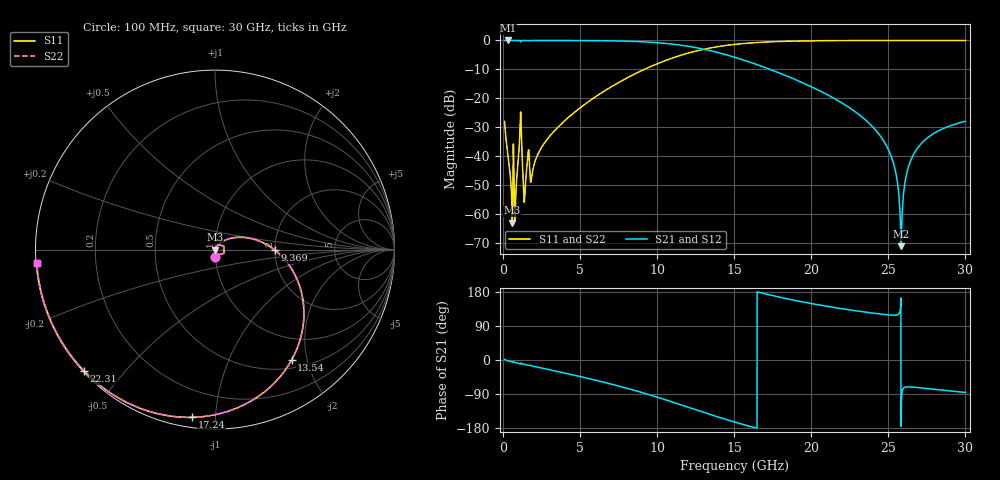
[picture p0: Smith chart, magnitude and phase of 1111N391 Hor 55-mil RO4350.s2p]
# GHz S MA R 50
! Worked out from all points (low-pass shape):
!   3201 points, 100 MHz to 30 GHz, reference 50 ohm
!   highest |S21| = 0.00 dB at 305.6 MHz (marker M1); lowest = -71.2 dB at 25.83 GHz (marker M2)
!   |S21| within 3 dB of the highest: start of sweep to 13 GHz
!   lowest |S11| = -63.1 dB at 595.2 MHz (marker M3), VSWR 1.00, Z = 50.1 - j0.0355 ohm
!   |S11| at or under -10 dB: start of sweep to 9.173 GHz
!   |S22| runs from -63.1 to 0.0 dB; largest |S21 - S12| = 0
!   S11 on the Smith chart (normalised r, x): 100 MHz: 1.00, -0.08; 9.369 GHz: 2.00, -0.01; 13.54 GHz: 0.62, -1.74; 17.24 GHz: 0.05, -0.87; 22.31 GHz: 0.00, -0.39; 30 GHz: 0.00, -0.04
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0.1  0.03985 -88.2  0.9989 1.5  0.9989 1.5  0.03985 -88.2
0.3055625  0.01083 -90.0  0.9995 -1.9  0.9995 -1.9  0.01083 -90.0
0.5952188  0.0006979 -30.5  0.9993 -4.8  0.9993 -4.8  0.0006979 -30.5
0.8661875  0.003414 69.9  0.9991 -7.3  0.9991 -7.3  0.003414 69.9
1.099781  0.02979 54.7  0.987 -10.5  0.987 -10.5  0.02979 54.7
1.417469  0.002259 36.9  0.9983 -11.6  0.9983 -11.6  0.002259 36.9
1.604344  0.01011 46.7  0.9948 -13.6  0.9948 -13.6  0.01011 46.7
1.875312  0.004699 52.9  0.998 -15.5  0.998 -15.5  0.004699 52.9
2.781656  0.0182 63.3  0.9985 -23.5  0.9985 -23.5  0.0182 63.3
5.089563  0.07116 44.5  0.9956 -44.4  0.9956 -44.4  0.07116 44.5
9.369  0.334 -0.5  0.9391 -90.1  0.9391 -90.1  0.334 -0.5
10.06978  0.4013 -9.2  0.9121 -98.9  0.9121 -98.9  0.4013 -9.2
13.53631  0.7488 -55.2  0.6569 -144.9  0.6569 -144.9  0.7488 -55.2
15.05  0.8559 -74.2  0.51 -163.9  0.51 -163.9  0.8559 -74.2
17.23644  0.9433 -97.8  0.3222 172.5  0.3222 172.5  0.9433 -97.8
20.03956  0.9849 -121.6  0.1563 148.7  0.1563 148.7  0.9849 -121.6
22.31009  0.9947 -137.1  0.07325 133.4  0.07325 133.4  0.9947 -137.1
25.01978  0.9973 -152.5  0.01259 119.0  0.01259 119.0  0.9973 -152.5
25.83269  0.9974 -156.6  0.0002753 -147.7  0.0002753 -147.7  0.9974 -156.6
26.22512  0.9974 -158.6  0.005439 -71.2  0.005439 -71.2  0.9974 -158.6
26.85116  0.9973 -161.6  0.01319 -72.5  0.01319 -72.5  0.9973 -161.6
30  0.9965 -175.6  0.03982 -85.7  0.03982 -85.7  0.9965 -175.6
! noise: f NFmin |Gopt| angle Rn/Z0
0.1  0.0006706  0.7361  0.9255  0.0005079
3.417  0.008613  0.4328  26.89  0.002391
6.743  0.01511  0.4058  48.9  0.003537
10.06  0.02375  0.46  66.85  0.005456
13.39  0.03811  0.5748  84.37  0.009456
16.7  0.06755  0.7244  104  0.01923
20.03  0.1451  0.8612  124.6  0.04943
23.35  0.4803  0.9555  143.7  0.2366
26.67  2.022  0.9887  160.7  1.193
30  0.5957  0.9608  175.6  0.006544
